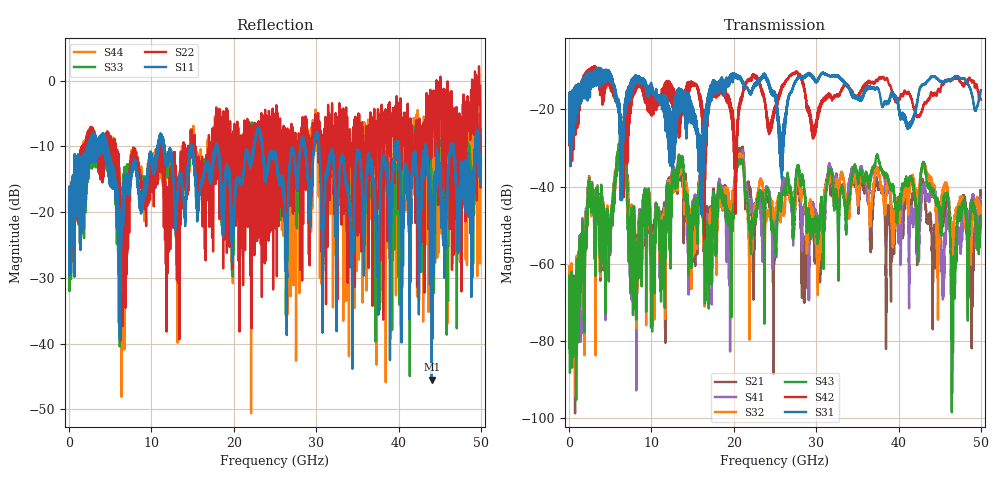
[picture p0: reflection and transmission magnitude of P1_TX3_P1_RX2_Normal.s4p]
!Keysight Technologies,N5225B,MY57041031,A.13.20.10
!Date: Friday, May 31, 2019 11:15:36
!Correction: S11(Full 4 Port(1,2,3,4))
!S12(Full 4 Port(1,2,3,4))
!S13(Full 4 Port(1,2,3,4))
!S14(Full 4 Port(1,2,3,4))
!S21(Full 4 Port(1,2,3,4))
!S22(Full 4 Port(1,2,3,4))
!S23(Full 4 Port(1,2,3,4))
!S24(Full 4 Port(1,2,3,4))
!S31(Full 4 Port(1,2,3,4))
!S32(Full 4 Port(1,2,3,4))
!S33(Full 4 Port(1,2,3,4))
!S34(Full 4 Port(1,2,3,4))
!S41(Full 4 Port(1,2,3,4))
!S42(Full 4 Port(1,2,3,4))
!S43(Full 4 Port(1,2,3,4))
!S44(Full 4 Port(1,2,3,4))
!S4P File: Measurements: <S11,S12,S13,S14>,
!<S21,S22,S23,S24>,
!<S31,S32,S33,S34>,
!<S41,S42,S43,S44>:
# Hz S  dB  R 50.0
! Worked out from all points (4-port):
!   5000 points, 10 MHz to 50 GHz, reference 50 ohm
!   strongest paths, dB at 10 MHz, 12.51 GHz, 25.01 GHz, 37.51 GHz, 50 GHz:
!     S31: -19.4, -27.2, -15.7, -14.6, -15.0
!     S42: -19.4, -16.4, -19.1, -12.6, -17.5
!     S43: -63.1, -40.1, -54.7, -32.4, -47.4
!     S32: -60.7, -38.7, -47.3, -37.2, -46.5
!     S41: -69.7, -38.2, -47.5, -36.4, -44.3
!     S21: -76.6, -36.8, -53.1, -40.8, -41.4
!   lowest |S11| = -45.5 dB at 44.03 GHz (marker M1), VSWR 1.01, Z = 50.1 + j0.527 ohm
!   |S11| at or under -10 dB: 4.66 GHz to 10.77 GHz (6.106 GHz wide, 79.2 % of centre); 23.49 GHz to 28.08 GHz (4.586 GHz wide, 17.8 % of centre); 30.37 GHz to 39.62 GHz (9.242 GHz wide, 26.4 % of centre)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
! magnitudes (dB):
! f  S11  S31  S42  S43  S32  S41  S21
! 10 MHz  -19.4  -19.4  -19.4  -63.1  -60.7  -69.7  -76.6
! 6.28 GHz  -26.0  -43.6  -27.7  -31.3  -30.7  -31.1  -30.8
! 10.15 GHz  -12.9  -14.3  -20.2  -60.0  -65.4  -76.1  -54.9
! 13.53 GHz  -14.1  -15.9  -19.5  -33.0  -34.3  -33.3  -34.9
! 17.12 GHz  -14.7  -14.6  -17.6  -54.5  -50.1  -51.0  -47.6
! 44.03 GHz  -45.5  -11.4  -15.8  -40.7  -38.7  -42.7  -55.2
! 50 GHz  -12.3  -15.0  -17.5  -47.4  -46.5  -44.3  -41.4
